PROGRAM P_Prog4
VAR

	fbKL6401 					: FB_LON_KL6401;

	fbREAD_094		: FB_READ_094_SNVT_preset;
	fbSEND_094		: FB_SEND_094_SNVT_preset;

	fbREAD_095		: FB_READ_095_SNVT_switch;
	fbSEND_095		: FB_SEND_095_SNVT_switch;

	fbREAD_096		: FB_READ_096_SNVT_trans_table;
	fbSEND_096		: FB_SEND_096_SNVT_trans_table;

	fbREAD_097		: FB_READ_097_SNVT_override;
	fbSEND_097		: FB_SEND_097_SNVT_override;

	fbREAD_098		: FB_READ_098_SNVT_pwr_fact;
	fbSEND_098		: FB_SEND_098_SNVT_pwr_fact;

	fbREAD_099		: FB_READ_099_SNVT_pwr_fact_f;
	fbSEND_099		: FB_SEND_099_SNVT_pwr_fact_f;

	fbREAD_100		: FB_READ_100_SNVT_density;
	fbSEND_100		: FB_SEND_100_SNVT_density;

	fbREAD_101		: FB_READ_101_SNVT_density_f;
	fbSEND_101		: FB_SEND_101_SNVT_density_f;

	fbREAD_102		: FB_READ_102_SNVT_rpm;
	fbSEND_102		: FB_SEND_102_SNVT_rpm;

	fbREAD_103		: FB_READ_103_SNVT_hvac_emerg;
	fbSEND_103		: FB_SEND_103_SNVT_hvac_emerg;

	fbREAD_104		: FB_READ_104_SNVT_angle_deg;
	fbSEND_104		: FB_SEND_104_SNVT_angle_deg;

	fbREAD_105		: FB_READ_105_SNVT_temp_p;
	fbSEND_105		: FB_SEND_105_SNVT_temp_p;

	fbREAD_106		: FB_READ_106_SNVT_temp_setpt;
	fbSEND_106		: FB_SEND_106_SNVT_temp_setpt;

	fbREAD_107		: FB_READ_107_SNVT_time_sec;
	fbSEND_107		: FB_SEND_107_SNVT_time_sec;

	fbREAD_108		: FB_READ_108_SNVT_hvac_mode;
	fbSEND_108		: FB_SEND_108_SNVT_hvac_mode;

	fbREAD_109		: FB_READ_109_SNVT_occupancy;
	fbSEND_109		: FB_SEND_109_SNVT_occupancy;

	fbREAD_110		: FB_READ_110_SNVT_area;
	fbSEND_110		: FB_SEND_110_SNVT_area;

	fbREAD_111		: FB_READ_111_SNVT_hvac_overid;
	fbSEND_111		: FB_SEND_111_SNVT_hvac_overid;

	fbREAD_112		: FB_READ_112_SNVT_hvac_status;
	fbSEND_112		: FB_SEND_112_SNVT_hvac_status;

	fbREAD_113		: FB_READ_113_SNVT_press_p;
	fbSEND_113		: FB_SEND_113_SNVT_press_p;

	fbREAD_114		: FB_READ_114_SNVT_address;
	fbSEND_114		: FB_SEND_114_SNVT_address;

	fbREAD_115		: FB_READ_115_SNVT_scene;
	fbSEND_115		: FB_SEND_115_SNVT_scene;

	fbREAD_116		: FB_READ_116_SNVT_scene_cfg;
	fbSEND_116		: FB_SEND_116_SNVT_scene_cfg;

	fbREAD_117		: FB_READ_117_SNVT_setting;
	fbSEND_117		: FB_SEND_117_SNVT_setting;

	fbREAD_118		: FB_READ_118_SNVT_evap_state;
	fbSEND_118		: FB_SEND_118_SNVT_evap_state;

	fbREAD_119		: FB_READ_119_SNVT_therm_mode;
	fbSEND_119		: FB_SEND_119_SNVT_therm_mode;

	fbREAD_120		: FB_READ_120_SNVT_defr_mode;
	fbSEND_120		: FB_SEND_120_SNVT_defr_mode;

	fbREAD_121		: FB_READ_121_SNVT_defr_term;
	fbSEND_121		: FB_SEND_121_SNVT_defr_term;

	fbREAD_122		: FB_READ_122_SNVT_defr_state;
	fbSEND_122		: FB_SEND_122_SNVT_defr_state;

	fbREAD_123		: FB_READ_123_SNVT_time_min;
	fbSEND_123		: FB_SEND_123_SNVT_time_min;

	fbREAD_124		: FB_READ_124_SNVT_time_hour;
	fbSEND_124		: FB_SEND_124_SNVT_time_hour;

END_VAR

fbKL6401(
	bDisabled:=FALSE ,
	stParameter_IN:=LON_IN_4 ,
	stParameter_OUT:=LON_OUT_4 ,
	stLON_Com:=stLON_Com_4,
	bReady=> ,
	eError=> ,
	stKL6401=> ,
	arrProgID=> ,
	arrNeuronID=> ,
	bBusy=> ,
	bError=> ,
	dwErrorKL=> ,
	bTimeOut=> ,
	byLONState=> );

(**)
fbREAD_094(
	wNVIndex:=0 ,
	bDisabled:= ,
	stLON_Com:=stLON_Com_4,
	stValue=> ,
	bNewData=> ,
	bError=> ,
	eError=> );
fbREAD_094.stValue;
fbREAD_094.bError;
fbREAD_094.eError;

fbSEND_094.stValue;
fbSEND_094.bStart;
fbSEND_094.bError;
fbSEND_094.eError;
fbSEND_094.bBusy;
fbSEND_094.dwErrorKL;

fbSEND_094.bAuto;
fbSEND_094.bSendInit;
fbSEND_094.tMinSendTime;
fbSEND_094.tMaxSendTime;

fbSEND_094(
	wNVIndex:=1 ,
	bStart:= ,
	stValue:= ,
	bDisabled:= ,
	stLON_Com:=stLON_Com_4,
	bError=> ,
	eError=> );
fbSEND_094.bStart:=FALSE;


(**)
fbREAD_095(
	wNVIndex:=2 ,
	bDisabled:= ,
	stLON_Com:=stLON_Com_4,
	stValue=> ,
	bNewData=> ,
	bError=> ,
	eError=> );
fbREAD_095.stValue;
fbREAD_095.bError;
fbREAD_095.eError;

fbSEND_095.stValue;
fbSEND_095.bStart;
fbSEND_095.bError;
fbSEND_095.eError;
fbSEND_095.bBusy;
fbSEND_095.dwErrorKL;

fbSEND_095.bAuto;
fbSEND_095.bSendInit;
fbSEND_095.tMinSendTime;
fbSEND_095.tMaxSendTime;

fbSEND_095(
	wNVIndex:=3 ,
	bStart:= ,
	stValue:= ,
	bDisabled:= ,
	stLON_Com:=stLON_Com_4,
	bError=> ,
	eError=> );
fbSEND_095.bStart:=FALSE;

(**)
fbREAD_096(
	wNVIndex:=4 ,
	bDisabled:= ,
	stLON_Com:=stLON_Com_4,
	stValue=> ,
	bNewData=> ,
	bError=> ,
	eError=> );
fbREAD_096.stValue;
fbREAD_096.bError;
fbREAD_096.eError;

fbSEND_096.stValue;
fbSEND_096.bStart;
fbSEND_096.bError;
fbSEND_096.eError;
fbSEND_096.bBusy;
fbSEND_096.dwErrorKL;


fbSEND_096.bAuto;
fbSEND_096.bSendInit;
fbSEND_096.tMinSendTime;
fbSEND_096.tMaxSendTime;

fbSEND_096(
	wNVIndex:=5 ,
	bStart:= ,
	stValue:= ,
	bDisabled:= ,
	stLON_Com:=stLON_Com_4,
	bError=> ,
	eError=> );
fbSEND_096.bStart:=FALSE;

(**)
fbREAD_097(
	wNVIndex:=6 ,
	bDisabled:= ,
	stLON_Com:=stLON_Com_4,
	eValue=> ,
	bNewData=> ,
	bError=> ,
	eError=> );
fbREAD_097.eValue;
fbREAD_097.bError;
fbREAD_097.eError;

fbSEND_097.eValue;
fbSEND_097.bStart;
fbSEND_097.bError;
fbSEND_097.eError;
fbSEND_097.bBusy;
fbSEND_097.dwErrorKL;

fbSEND_097.bAuto;
fbSEND_097.bSendInit;
fbSEND_097.tMinSendTime;
fbSEND_097.tMaxSendTime;

fbSEND_097(
	wNVIndex:=7 ,
	bStart:= ,
	eValue:= ,
	bDisabled:= ,
	stLON_Com:=stLON_Com_4,
	bError=> ,
	eError=> );
fbSEND_097.bStart:=FALSE;

(**)
fbREAD_098(
	wNVIndex:=8 ,
	bDisabled:= ,
	stLON_Com:=stLON_Com_4,
	rValue=> ,
	bNewData=> ,
	bError=> ,
	eError=> );
fbREAD_098.rValue;
fbREAD_098.bError;
fbREAD_098.eError;

fbSEND_098.rValue;
fbSEND_098.bStart;
fbSEND_098.bError;
fbSEND_098.eError;
fbSEND_098.bBusy;
fbSEND_098.dwErrorKL;

fbSEND_098.bAuto;
fbSEND_098.bSendInit;
fbSEND_098.tMinSendTime;
fbSEND_098.tMaxSendTime;
fbSEND_098.rValueLimit;

fbSEND_098(
	wNVIndex:=9 ,
	bStart:= ,
	rValue:= ,
	bDisabled:= ,
	stLON_Com:=stLON_Com_4,
	bError=> ,
	eError=> );
fbSEND_098.bStart:=FALSE;

(**)
fbREAD_099(
	wNVIndex:=10 ,
	bDisabled:= ,
	stLON_Com:=stLON_Com_4,
	rValue=> ,
	bNewData=> ,
	bError=> ,
	eError=> );
fbREAD_099.rValue;
fbREAD_099.bError;
fbREAD_099.eError;

fbSEND_099.rValue;
fbSEND_099.bStart;
fbSEND_099.bError;
fbSEND_099.eError;
fbSEND_099.bBusy;
fbSEND_099.dwErrorKL;

fbSEND_099.bAuto;
fbSEND_099.bSendInit;
fbSEND_099.tMinSendTime;
fbSEND_099.tMaxSendTime;
fbSEND_099.rValueLimit;

fbSEND_099(
	wNVIndex:=11 ,
	bStart:= ,
	rValue:= ,
	bDisabled:= ,
	stLON_Com:=stLON_Com_4,
	bError=> ,
	eError=> );
fbSEND_099.bStart:=FALSE;

(**)
fbREAD_100(
	wNVIndex:=12 ,
	bDisabled:= ,
	stLON_Com:=stLON_Com_4,
	rValue=> ,
	bNewData=> ,
	bError=> ,
	eError=> );
fbREAD_100.rValue;
fbREAD_100.bError;
fbREAD_100.eError;

fbSEND_100.rValue;
fbSEND_100.bStart;
fbSEND_100.bError;
fbSEND_100.eError;
fbSEND_100.bBusy;
fbSEND_100.dwErrorKL;

fbSEND_100.bAuto;
fbSEND_100.bSendInit;
fbSEND_100.tMinSendTime;
fbSEND_100.tMaxSendTime;
fbSEND_100.rValueLimit;

fbSEND_100(
	wNVIndex:=13 ,
	bStart:= ,
	rValue:= ,
	bDisabled:= ,
	stLON_Com:=stLON_Com_4,
	bError=> ,
	eError=> );
fbSEND_100.bStart:=FALSE;

(**)
fbREAD_101(
	wNVIndex:=14 ,
	bDisabled:= ,
	stLON_Com:=stLON_Com_4,
	rValue=> ,
	bNewData=> ,
	bError=> ,
	eError=> );
fbREAD_101.rValue;
fbREAD_101.bError;
fbREAD_101.eError;

fbSEND_101.rValue;
fbSEND_101.bStart;
fbSEND_101.bError;
fbSEND_101.eError;
fbSEND_101.bBusy;
fbSEND_101.dwErrorKL;

fbSEND_101.bAuto;
fbSEND_101.bSendInit;
fbSEND_101.tMinSendTime;
fbSEND_101.tMaxSendTime;
fbSEND_101.rValueLimit;

fbSEND_101(
	wNVIndex:=15 ,
	bStart:= ,
	rValue:= ,
	bDisabled:= ,
	stLON_Com:=stLON_Com_4,
	bError=> ,
	eError=> );
fbSEND_101.bStart:=FALSE;

(**)
fbREAD_102(
	wNVIndex:=16 ,
	bDisabled:= ,
	stLON_Com:=stLON_Com_4,
	uiValue=> ,
	bNewData=> ,
	bError=> ,
	eError=> );
fbREAD_102.uiValue;
fbREAD_102.bError;
fbREAD_102.eError;

fbSEND_102.uiValue;
fbSEND_102.bStart;
fbSEND_102.bError;
fbSEND_102.eError;
fbSEND_102.bBusy;
fbSEND_102.dwErrorKL;

fbSEND_102.bAuto;
fbSEND_102.bSendInit;
fbSEND_102.tMinSendTime;
fbSEND_102.tMaxSendTime;
fbSEND_102.uiValueLimit;

fbSEND_102(
	wNVIndex:=17 ,
	bStart:= ,
	uiValue:= ,
	bDisabled:= ,
	stLON_Com:=stLON_Com_4,
	bError=> ,
	eError=> );
fbSEND_102.bStart:=FALSE;

(**)
fbREAD_103(
	wNVIndex:=18 ,
	bDisabled:= ,
	stLON_Com:=stLON_Com_4,
	eValue=> ,
	bNewData=> ,
	bError=> ,
	eError=> );
fbREAD_103.eValue;
fbREAD_103.bError;
fbREAD_103.eError;

fbSEND_103.eValue;
fbSEND_103.bStart;
fbSEND_103.bError;
fbSEND_103.eError;
fbSEND_103.bBusy;
fbSEND_103.dwErrorKL;

fbSEND_103.bAuto;
fbSEND_103.bSendInit;
fbSEND_103.tMinSendTime;
fbSEND_103.tMaxSendTime;

fbSEND_103(
	wNVIndex:=19 ,
	bStart:= ,
	eValue:= ,
	bDisabled:= ,
	stLON_Com:=stLON_Com_4,
	bError=> ,
	eError=> );
fbSEND_103.bStart:=FALSE;

(**)
fbREAD_104(
	wNVIndex:=20 ,
	bDisabled:= ,
	stLON_Com:=stLON_Com_4,
	rValue=> ,
	bNewData=> ,
	bError=> ,
	eError=> );
fbREAD_104.rValue;
fbREAD_104.bError;
fbREAD_104.eError;

fbSEND_104.rValue;
fbSEND_104.bStart;
fbSEND_104.bError;
fbSEND_104.eError;
fbSEND_104.bBusy;
fbSEND_104.dwErrorKL;

fbSEND_104.bAuto;
fbSEND_104.bSendInit;
fbSEND_104.tMinSendTime;
fbSEND_104.tMaxSendTime;
fbSEND_104.rValueLimit;

fbSEND_104(
	wNVIndex:=21 ,
	bStart:= ,
	rValue:= ,
	bDisabled:= ,
	stLON_Com:=stLON_Com_4,
	bError=> ,
	eError=> );
fbSEND_104.bStart:=FALSE;

(**)
fbREAD_105(
	wNVIndex:=22 ,
	bDisabled:= ,
	stLON_Com:=stLON_Com_4,
	rValue=> ,
	bNewData=> ,
	bError=> ,
	eError=> );
fbREAD_105.rValue;
fbREAD_105.bError;
fbREAD_105.eError;

fbSEND_105.rValue;
fbSEND_105.bStart;
fbSEND_105.bError;
fbSEND_105.eError;
fbSEND_105.bBusy;
fbSEND_105.dwErrorKL;

fbSEND_105.bAuto;
fbSEND_105.bSendInit;
fbSEND_105.tMinSendTime;
fbSEND_105.tMaxSendTime;

fbSEND_105(
	wNVIndex:=23 ,
	bStart:= ,
	rValue:= ,
	bDisabled:= ,
	stLON_Com:=stLON_Com_4,
	bError=> ,
	eError=> );
fbSEND_105.bStart:=FALSE;

(**)
fbREAD_106(
	wNVIndex:=24 ,
	bDisabled:= ,
	stLON_Com:=stLON_Com_4,
	stValue=> ,
	bNewData=> ,
	bError=> ,
	eError=> );
fbREAD_106.stValue;
fbREAD_106.bError;
fbREAD_106.eError;

fbSEND_106.stValue;
fbSEND_106.bStart;
fbSEND_106.bError;
fbSEND_106.eError;
fbSEND_106.bBusy;
fbSEND_106.dwErrorKL;

fbSEND_106.bAuto;
fbSEND_106.bSendInit;
fbSEND_106.tMinSendTime;
fbSEND_106.tMaxSendTime;

fbSEND_106(
	wNVIndex:=25 ,
	bStart:= ,
	stValue:= ,
	bDisabled:= ,
	stLON_Com:=stLON_Com_4,
	bError=> ,
	eError=> );
fbSEND_106.bStart:=FALSE;

(**)
fbREAD_107(
	wNVIndex:=26 ,
	bDisabled:= ,
	stLON_Com:=stLON_Com_4,
	rValue=> ,
	bNewData=> ,
	bError=> ,
	eError=> );
fbREAD_107.rValue;
fbREAD_107.bError;
fbREAD_107.eError;

fbSEND_107.rValue;
fbSEND_107.bStart;
fbSEND_107.bError;
fbSEND_107.eError;
fbSEND_107.bBusy;
fbSEND_107.dwErrorKL;

fbSEND_107.bAuto;
fbSEND_107.bSendInit;
fbSEND_107.tMinSendTime;
fbSEND_107.tMaxSendTime;
fbSEND_107.rValueLimit;

fbSEND_107(
	wNVIndex:=27 ,
	bStart:= ,
	rValue:= ,
	bDisabled:= ,
	stLON_Com:=stLON_Com_4,
	bError=> ,
	eError=> );
fbSEND_107.bStart:=FALSE;

(**)
fbREAD_108(
	wNVIndex:=28 ,
	bDisabled:= ,
	stLON_Com:=stLON_Com_4,
	eValue=> ,
	bNewData=> ,
	bError=> ,
	eError=> );
fbREAD_108.eValue;
fbREAD_108.bError;
fbREAD_108.eError;

fbSEND_108.eValue;
fbSEND_108.bStart;
fbSEND_108.bError;
fbSEND_108.eError;
fbSEND_108.bBusy;
fbSEND_108.dwErrorKL;

fbSEND_108.bAuto;
fbSEND_108.bSendInit;
fbSEND_108.tMinSendTime;
fbSEND_108.tMaxSendTime;

fbSEND_108(
	wNVIndex:=29 ,
	bStart:= ,
	eValue:= ,
	bDisabled:= ,
	stLON_Com:=stLON_Com_4,
	bError=> ,
	eError=> );
fbSEND_108.bStart:=FALSE;

(**)
fbREAD_109(
	wNVIndex:=30 ,
	bDisabled:= ,
	stLON_Com:=stLON_Com_4,
	eValue=> ,
	bNewData=> ,
	bError=> ,
	eError=> );
fbREAD_109.eValue;
fbREAD_109.bError;
fbREAD_109.eError;

fbSEND_109.eValue;
fbSEND_109.bStart;
fbSEND_109.bError;
fbSEND_109.eError;
fbSEND_109.bBusy;
fbSEND_109.dwErrorKL;

fbSEND_109.bAuto;
fbSEND_109.bSendInit;
fbSEND_109.tMinSendTime;
fbSEND_109.tMaxSendTime;

fbSEND_109(
	wNVIndex:=31 ,
	bStart:= ,
	eValue:= ,
	bDisabled:= ,
	stLON_Com:=stLON_Com_4,
	bError=> ,
	eError=> );
fbSEND_109.bStart:=FALSE;

(**)
fbREAD_110(
	wNVIndex:=32 ,
	bDisabled:= ,
	stLON_Com:=stLON_Com_4,
	rValue=> ,
	bNewData=> ,
	bError=> ,
	eError=> );
fbREAD_110.rValue;
fbREAD_110.bError;
fbREAD_110.eError;

fbSEND_110.rValue;
fbSEND_110.bStart;
fbSEND_110.bError;
fbSEND_110.eError;
fbSEND_110.bBusy;
fbSEND_110.dwErrorKL;

fbSEND_110.bAuto;
fbSEND_110.bSendInit;
fbSEND_110.tMinSendTime;
fbSEND_110.tMaxSendTime;
fbSEND_110.rValueLimit;

fbSEND_110(
	wNVIndex:=33 ,
	bStart:= ,
	rValue:= ,
	bDisabled:= ,
	stLON_Com:=stLON_Com_4,
	bError=> ,
	eError=> );
fbSEND_110.bStart:=FALSE;

(**)
fbREAD_111(
	wNVIndex:=34 ,
	bDisabled:= ,
	stLON_Com:=stLON_Com_4,
	stValue=> ,
	bNewData=> ,
	bError=> ,
	eError=> );
fbREAD_111.stValue;
fbREAD_111.bError;
fbREAD_111.eError;

fbSEND_111.stValue;
fbSEND_111.bStart;
fbSEND_111.bError;
fbSEND_111.eError;
fbSEND_111.bBusy;
fbSEND_111.dwErrorKL;

fbSEND_111.bAuto;
fbSEND_111.bSendInit;
fbSEND_111.tMinSendTime;
fbSEND_111.tMaxSendTime;

fbSEND_111(
	wNVIndex:=35 ,
	bStart:= ,
	stValue:= ,
	bDisabled:= ,
	stLON_Com:=stLON_Com_4,
	bError=> ,
	eError=> );
fbSEND_111.bStart:=FALSE;

(**)
fbREAD_112(
	wNVIndex:=36 ,
	bDisabled:= ,
	stLON_Com:=stLON_Com_4,
	stValue=> ,
	bNewData=> ,
	bError=> ,
	eError=> );
fbREAD_112.stValue;
fbREAD_112.bError;
fbREAD_112.eError;

fbSEND_112.stValue;
fbSEND_112.bStart;
fbSEND_112.bError;
fbSEND_112.eError;
fbSEND_112.bBusy;
fbSEND_112.dwErrorKL;

fbSEND_112.bAuto;
fbSEND_112.bSendInit;
fbSEND_112.tMinSendTime;
fbSEND_112.tMaxSendTime;

fbSEND_112(
	wNVIndex:=37 ,
	bStart:= ,
	stValue:= ,
	bDisabled:= ,
	stLON_Com:=stLON_Com_4,
	bError=> ,
	eError=> );
fbSEND_112.bStart:=FALSE;

(**)
fbREAD_113(
	wNVIndex:=38 ,
	bDisabled:= ,
	stLON_Com:=stLON_Com_4,
	iValue=> ,
	bNewData=> ,
	bError=> ,
	eError=> );
fbREAD_113.iValue;
fbREAD_113.bError;
fbREAD_113.eError;

fbSEND_113.iValue;
fbSEND_113.bStart;
fbSEND_113.bError;
fbSEND_113.eError;
fbSEND_113.bBusy;
fbSEND_113.dwErrorKL;

fbSEND_113.bAuto;
fbSEND_113.bSendInit;
fbSEND_113.tMinSendTime;
fbSEND_113.tMaxSendTime;
fbSEND_113.iValueLimit;

fbSEND_113(
	wNVIndex:=39 ,
	bStart:= ,
	iValue:= ,
	bDisabled:= ,
	stLON_Com:=stLON_Com_4,
	bError=> ,
	eError=> );
fbSEND_113.bStart:=FALSE;

(**)
fbREAD_114(
	wNVIndex:=40 ,
	bDisabled:= ,
	stLON_Com:=stLON_Com_4,
	uiValue=> ,
	bNewData=> ,
	bError=> ,
	eError=> );
fbREAD_114.uiValue;
fbREAD_114.bError;
fbREAD_114.eError;

fbSEND_114.uiValue;
fbSEND_114.bStart;
fbSEND_114.bError;
fbSEND_114.eError;
fbSEND_114.bBusy;
fbSEND_114.dwErrorKL;

fbSEND_114.bAuto;
fbSEND_114.bSendInit;
fbSEND_114.tMinSendTime;
fbSEND_114.tMaxSendTime;
fbSEND_114.uiValueLimit;

fbSEND_114(
	wNVIndex:=41 ,
	bStart:= ,
	uiValue:= ,
	bDisabled:= ,
	stLON_Com:=stLON_Com_4,
	bError=> ,
	eError=> );
fbSEND_114.bStart:=FALSE;

(**)
fbREAD_115(
	wNVIndex:=42 ,
	bDisabled:= ,
	stLON_Com:=stLON_Com_4,
	stValue=> ,
	bNewData=> ,
	bError=> ,
	eError=> );
fbREAD_115.stValue;
fbREAD_115.bError;
fbREAD_115.eError;

fbSEND_115.stValue;
fbSEND_115.bStart;
fbSEND_115.bError;
fbSEND_115.eError;
fbSEND_115.bBusy;
fbSEND_115.dwErrorKL;

fbSEND_115.bAuto;
fbSEND_115.bSendInit;
fbSEND_115.tMinSendTime;
fbSEND_115.tMaxSendTime;

fbSEND_115(
	wNVIndex:=43 ,
	bStart:= ,
	stValue:= ,
	bDisabled:= ,
	stLON_Com:=stLON_Com_4,
	bError=> ,
	eError=> );
fbSEND_115.bStart:=FALSE;

(**)
fbREAD_116(
	wNVIndex:=44 ,
	bDisabled:= ,
	stLON_Com:=stLON_Com_4,
	stValue=> ,
	bNewData=> ,
	bError=> ,
	eError=> );
fbREAD_116.stValue;
fbREAD_116.bError;
fbREAD_116.eError;

fbSEND_116.stValue;
fbSEND_116.bStart;
fbSEND_116.bError;
fbSEND_116.eError;
fbSEND_116.bBusy;
fbSEND_116.dwErrorKL;

fbSEND_116.bAuto;
fbSEND_116.bSendInit;
fbSEND_116.tMinSendTime;
fbSEND_116.tMaxSendTime;

fbSEND_116(
	wNVIndex:=45 ,
	bStart:= ,
	stValue:= ,
	bDisabled:= ,
	stLON_Com:=stLON_Com_4,
	bError=> ,
	eError=> );
fbSEND_116.bStart:=FALSE;

(**)
fbREAD_117(
	wNVIndex:=46 ,
	bDisabled:= ,
	stLON_Com:=stLON_Com_4,
	stValue=> ,
	bNewData=> ,
	bError=> ,
	eError=> );
fbREAD_117.stValue;
fbREAD_117.bError;
fbREAD_117.eError;

fbSEND_117.stValue;
fbSEND_117.bStart;
fbSEND_117.bError;
fbSEND_117.eError;
fbSEND_117.bBusy;
fbSEND_117.dwErrorKL;

fbSEND_117.bAuto;
fbSEND_117.bSendInit;
fbSEND_117.tMinSendTime;
fbSEND_117.tMaxSendTime;

fbSEND_117(
	wNVIndex:=47 ,
	bStart:= ,
	stValue:= ,
	bDisabled:= ,
	stLON_Com:=stLON_Com_4,
	bError=> ,
	eError=> );
fbSEND_117.bStart:=FALSE;

(**)
fbREAD_118(
	wNVIndex:=48 ,
	bDisabled:= ,
	stLON_Com:=stLON_Com_4,
	eValue=> ,
	bNewData=> ,
	bError=> ,
	eError=> );
fbREAD_118.eValue;
fbREAD_118.bError;
fbREAD_118.eError;

fbSEND_118.eValue;
fbSEND_118.bStart;
fbSEND_118.bError;
fbSEND_118.eError;
fbSEND_118.bBusy;
fbSEND_118.dwErrorKL;

fbSEND_118.bAuto;
fbSEND_118.bSendInit;
fbSEND_118.tMinSendTime;
fbSEND_118.tMaxSendTime;

fbSEND_118(
	wNVIndex:=49 ,
	bStart:= ,
	eValue:= ,
	bDisabled:= ,
	stLON_Com:=stLON_Com_4,
	bError=> ,
	eError=> );
fbSEND_118.bStart:=FALSE;

(**)
fbREAD_119(
	wNVIndex:=50 ,
	bDisabled:= ,
	stLON_Com:=stLON_Com_4,
	eValue=> ,
	bNewData=> ,
	bError=> ,
	eError=> );
fbREAD_119.eValue;
fbREAD_119.bError;
fbREAD_119.eError;

fbSEND_119.eValue;
fbSEND_119.bStart;
fbSEND_119.bError;
fbSEND_119.eError;
fbSEND_119.bBusy;
fbSEND_119.dwErrorKL;

fbSEND_119.bAuto;
fbSEND_119.bSendInit;
fbSEND_119.tMinSendTime;
fbSEND_119.tMaxSendTime;

fbSEND_119(
	wNVIndex:=51 ,
	bStart:= ,
	eValue:= ,
	bDisabled:= ,
	stLON_Com:=stLON_Com_4,
	bError=> ,
	eError=> );
fbSEND_119.bStart:=FALSE;


(**)
fbREAD_120(
	wNVIndex:=52 ,
	bDisabled:= ,
	stLON_Com:=stLON_Com_4,
	eValue=> ,
	bNewData=> ,
	bError=> ,
	eError=> );
fbREAD_120.eValue;
fbREAD_120.bError;
fbREAD_120.eError;

fbSEND_120.eValue;
fbSEND_120.bStart;
fbSEND_120.bError;
fbSEND_120.eError;
fbSEND_120.bBusy;
fbSEND_120.dwErrorKL;

fbSEND_120.bAuto;
fbSEND_120.bSendInit;
fbSEND_120.tMinSendTime;
fbSEND_120.tMaxSendTime;

fbSEND_120(
	wNVIndex:=53 ,
	bStart:= ,
	eValue:= ,
	bDisabled:= ,
	stLON_Com:=stLON_Com_4,
	bError=> ,
	eError=> );
fbSEND_120.bStart:=FALSE;

(**)
fbREAD_121(
	wNVIndex:=54 ,
	bDisabled:= ,
	stLON_Com:=stLON_Com_4,
	eValue=> ,
	bNewData=> ,
	bError=> ,
	eError=> );
fbREAD_121.eValue;
fbREAD_121.bError;
fbREAD_121.eError;

fbSEND_121.eValue;
fbSEND_121.bStart;
fbSEND_121.bError;
fbSEND_121.eError;
fbSEND_121.bBusy;
fbSEND_121.dwErrorKL;

fbSEND_121.bAuto;
fbSEND_121.bSendInit;
fbSEND_121.tMinSendTime;
fbSEND_121.tMaxSendTime;

fbSEND_121(
	wNVIndex:=55 ,
	bStart:= ,
	eValue:= ,
	bDisabled:= ,
	stLON_Com:=stLON_Com_4,
	bError=> ,
	eError=> );
fbSEND_121.bStart:=FALSE;

(**)
fbREAD_122(
	wNVIndex:=56 ,
	bDisabled:= ,
	stLON_Com:=stLON_Com_4,
	eValue=> ,
	bNewData=> ,
	bError=> ,
	eError=> );
fbREAD_122.eValue;
fbREAD_122.bError;
fbREAD_122.eError;

fbSEND_122.eValue;
fbSEND_122.bStart;
fbSEND_122.bError;
fbSEND_122.eError;
fbSEND_122.bBusy;
fbSEND_122.dwErrorKL;

fbSEND_122.bAuto;
fbSEND_122.bSendInit;
fbSEND_122.tMinSendTime;
fbSEND_122.tMaxSendTime;

fbSEND_122(
	wNVIndex:=57 ,
	bStart:= ,
	eValue:= ,
	bDisabled:= ,
	stLON_Com:=stLON_Com_4,
	bError=> ,
	eError=> );
fbSEND_122.bStart:=FALSE;

(**)
fbREAD_123(
	wNVIndex:=58 ,
	bDisabled:= ,
	stLON_Com:=stLON_Com_4,
	uiValue=> ,
	bNewData=> ,
	bError=> ,
	eError=> );
fbREAD_123.uiValue;
fbREAD_123.bError;
fbREAD_123.eError;

fbSEND_123.uiValue;
fbSEND_123.bStart;
fbSEND_123.bError;
fbSEND_123.eError;
fbSEND_123.bBusy;
fbSEND_123.dwErrorKL;

fbSEND_123.bAuto;
fbSEND_123.bSendInit;
fbSEND_123.tMinSendTime;
fbSEND_123.tMaxSendTime;
fbSEND_123.uiValueLimit;

fbSEND_123(
	wNVIndex:=59 ,
	bStart:= ,
	uiValue:= ,
	bDisabled:= ,
	stLON_Com:=stLON_Com_4,
	bError=> ,
	eError=> );
fbSEND_123.bStart:=FALSE;

(**)
fbREAD_124(
	wNVIndex:=60 ,
	bDisabled:= ,
	stLON_Com:=stLON_Com_4,
	uiValue=> ,
	bNewData=> ,
	bError=> ,
	eError=> );
fbREAD_124.uiValue;
fbREAD_124.bError;
fbREAD_124.eError;

fbSEND_124.uiValue;
fbSEND_124.bStart;
fbSEND_124.bError;
fbSEND_124.eError;
fbSEND_124.bBusy;
fbSEND_124.dwErrorKL;

fbSEND_124.bAuto;
fbSEND_124.bSendInit;
fbSEND_124.tMinSendTime;
fbSEND_124.tMaxSendTime;

fbSEND_124(
	wNVIndex:=61 ,
	bStart:= ,
	uiValue:= ,
	bDisabled:= ,
	stLON_Com:=stLON_Com_4,
	bError=> ,
	eError=> );
fbSEND_124.bStart:=FALSE;

END_PROGRAM
